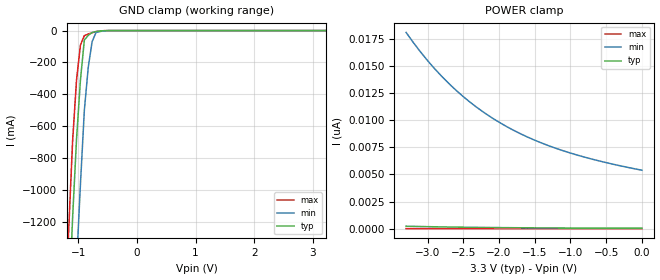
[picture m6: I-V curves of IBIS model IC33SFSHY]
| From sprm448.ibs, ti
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|   Model Cell IC33SFSHY
|IC33SFSHY
[Model]   IC33SFSHY
Model_type   Input
Polarity   Non-Inverting
Vinl =  0.8v
Vinh =  2v
C_comp   2.0027p   1.6434p   2.65p
[Model Spec]
Vinl   0.8v   0.8v   0.8v
Vinh   2v   2v   2v
[Temperature Range]   25   125   -40
[Voltage Range]   3.3   3   3.6
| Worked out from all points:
|   GND clamp passes 1 mA (typ) near -0.56 V on its own axis
[POWER_clamp]
|   voltage   I(typ)   I(min)   I(max)
-3.3V     227.6pA    18.09nA    4.636pA
-3.2V     212.4pA    17.17nA    4.352pA
-3V       185.4pA    15.5nA     3.713pA
-2.7V     151.7pA    13.37nA    2.718pA
-2.4V     125.2pA    11.63nA    2.203pA
-2.2V     110.4pA    10.66nA    1.998pA
-2V       97.98pA    9.816nA    1.616pA
-1.8V     87.28pA    9.082nA    1.332pA
-1.6V     78.02pA    8.443nA    1.164pA
-1.2V     63.46pA    7.399nA    1.03pA
-700mV    50.42pA    6.413nA    692.8fA
-11.55fV  37.64pA    5.387nA    430.8fA
[GND_clamp]
|   voltage   I(typ)   I(min)   I(max)
-3.3V     -22.4A     -23.17A    -21.98A
-1.233V   -2.327A    -3.192A    -1.823A
-1.167V   -1.741A    -2.598A    -1.245A
-1.1V     -1.17A     -2.014A    -689.7mA
-1.033V   -680.3mA   -1.468A    -310.1mA
-966.7mV  -310.1mA   -963.5mA   -90.79mA
-900mV    -59.58mA   -500mA     -31.71mA
-833.3mV  -29.85mA   -231.2mA   -21.86mA
-766.7mV  -12.04mA   -68.57mA   -13.38mA
-700mV    -6.164mA   -12.23mA   -6.285mA
-433.3mV  -64.46uA   -228.3uA   -21.14uA
3.233V    36.73pA    5.698nA    377.5fA
